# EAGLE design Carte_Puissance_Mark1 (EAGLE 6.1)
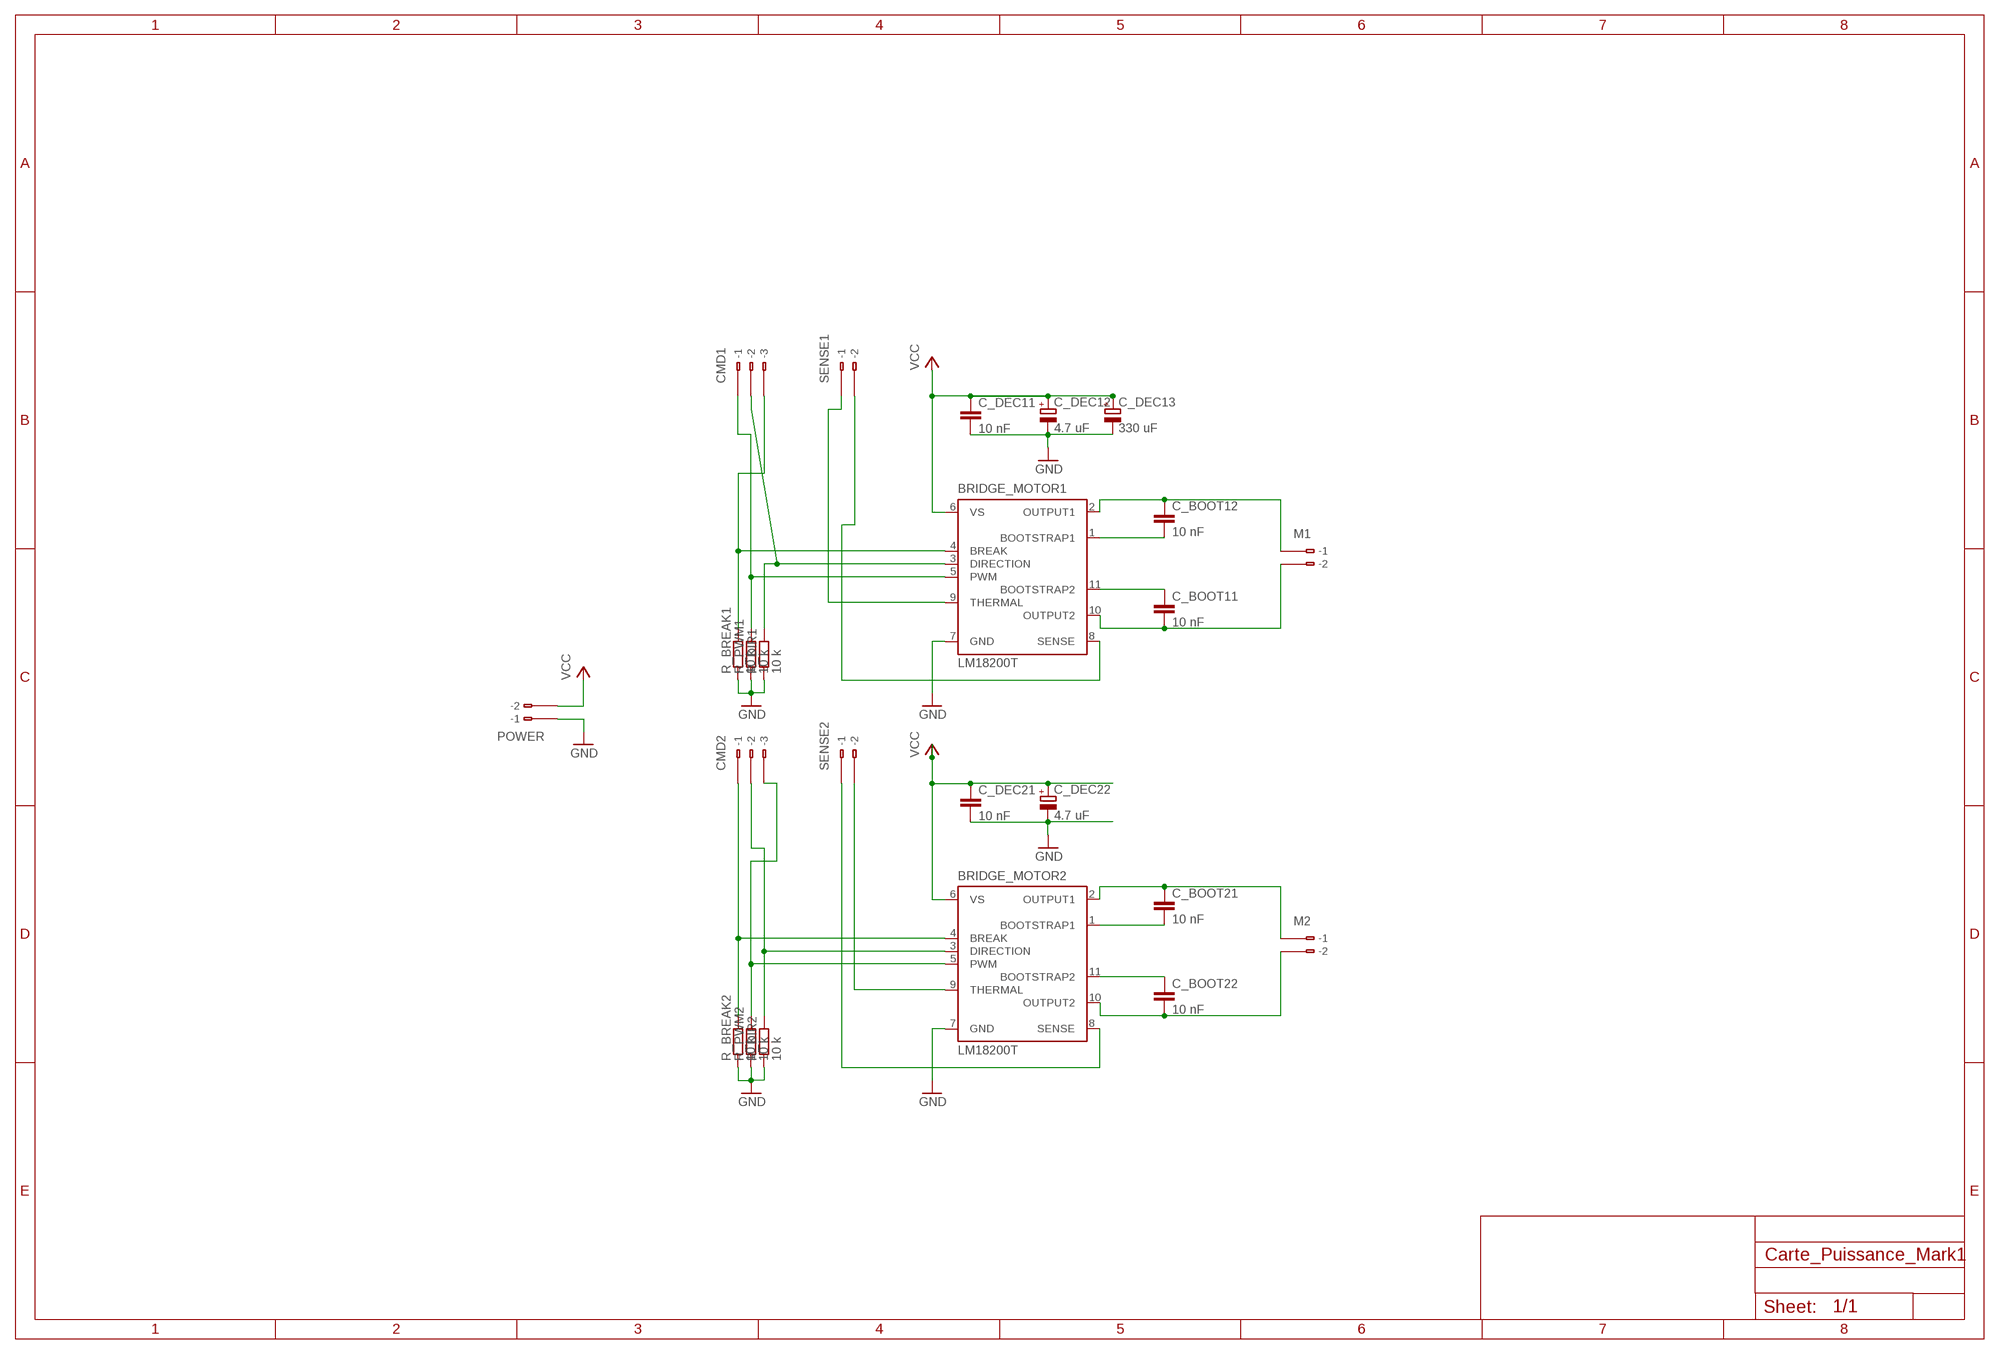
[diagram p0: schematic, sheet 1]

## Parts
BRIDGE_MOTOR1  LM18200T  [TO-220-11]
BRIDGE_MOTOR2  LM18200T  [TO-220-11]
C_BOOT11  10 nF  C5/3  [C5B3]
C_BOOT12  10 nF  C5/3  [C5B3]
C_BOOT21  10 nF  C5/3  [C5B3]
C_BOOT22  10 nF  C5/3  [C5B3]
C_DEC11  10 nF  C5/3  [C5B3]
C_DEC12  4.7 uF  CPOL-EUE2-5  [E2-5]
C_DEC13  330 uF  CPOL-EUE5-10.5  [E5-10,5]
C_DEC21  10 nF  C5/3  [C5B3]
C_DEC22  4.7 uF  CPOL-EUE2-5  [E2-5]
CMD1  233-103  [233-103]
CMD2  233-103  [233-103]
M1  233-102  [233-102]
M2  233-102  [233-102]
POWER  233-102  [233-102]
R_BREAK1  10 k  R-EU_R2012  [R2012]
R_BREAK2  10 k  R-EU_R2012  [R2012]
R_DIR1  10 k  R-EU_R2012  [R2012]
R_DIR2  10 k  R-EU_R2012  [R2012]
R_PWM1  10 k  R-EU_R2012  [R2012]
R_PWM2  10 k  R-EU_R2012  [R2012]
SENSE1  233-102  [233-102]
SENSE2  233-102  [233-102]

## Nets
GND: BRIDGE_MOTOR1.7(GND) BRIDGE_MOTOR2.7(GND) C_DEC11.2 C_DEC12.- C_DEC13.- C_DEC21.2 C_DEC22.- R_BREAK1.1 R_BREAK2.1 R_DIR1.1 R_DIR2.1 R_PWM1.1 R_PWM2.1
N$1: BRIDGE_MOTOR1.4(BREAK) CMD1.B3(B-3) R_BREAK1.2
N$2: BRIDGE_MOTOR1.5(PWM) CMD1.B1(B-1) R_PWM1.2
N$3: BRIDGE_MOTOR2.11(BOOTSTRAP2) C_BOOT22.1
N$4: BRIDGE_MOTOR2.1(BOOTSTRAP1) C_BOOT21.2
N$5: BRIDGE_MOTOR2.2(OUTPUT1) C_BOOT21.1 M2.B1(B-1)
N$6: BRIDGE_MOTOR2.10(OUTPUT2) C_BOOT22.2 M2.B2(B-2)
N$7: BRIDGE_MOTOR1.11(BOOTSTRAP2) C_BOOT11.1
N$8: BRIDGE_MOTOR1.1(BOOTSTRAP1) C_BOOT12.2
N$9: BRIDGE_MOTOR1.2(OUTPUT1) C_BOOT12.1 M1.B1(B-1)
N$10: BRIDGE_MOTOR1.10(OUTPUT2) C_BOOT11.2 M1.B2(B-2)
N$11: BRIDGE_MOTOR1.3(DIRECTION) CMD1.B2(B-2) R_DIR1.2
N$12: BRIDGE_MOTOR1.9(THERMAL) SENSE1.B1(B-1)
N$13: BRIDGE_MOTOR1.8(SENSE) SENSE1.B2(B-2)
N$14: BRIDGE_MOTOR2.4(BREAK) CMD2.B1(B-1) R_BREAK2.2
N$15: BRIDGE_MOTOR2.5(PWM) CMD2.B3(B-3) R_PWM2.2
N$16: BRIDGE_MOTOR2.3(DIRECTION) CMD2.B2(B-2) R_DIR2.2
N$17: BRIDGE_MOTOR2.9(THERMAL) SENSE2.B2(B-2)
N$18: BRIDGE_MOTOR2.8(SENSE) SENSE2.B1(B-1)
POWERT: POWER.B1(B-1) ; supply symbol labelled GND
VCC: BRIDGE_MOTOR1.6(VS) BRIDGE_MOTOR2.6(VS) C_DEC11.1 C_DEC12.+ C_DEC13.+ C_DEC21.1 C_DEC22.+ POWER.B2(B-2)
Unconnected: CMD1.A1(-1) CMD1.A2(-2) CMD1.A3(-3) CMD2.A1(-1) CMD2.A2(-2) CMD2.A3(-3) M1.A1(-1) M1.A2(-2) M2.A1(-1) M2.A2(-2) POWER.A1(-1) POWER.A2(-2) SENSE1.A1(-1) SENSE1.A2(-2) SENSE2.A1(-1) SENSE2.A2(-2)

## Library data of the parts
BRIDGE_MOTOR1 BRIDGE_MOTOR2 = national-semiconductor:LM18200T: 3A, 55V H-Bridge Motor Control SourcE: http://cache.national.com/ds/LM/LMD18200.pdf; OC_FARNELL: unknown; OC_NEWARK: unknown
C_BOOT11 C_BOOT12 C_BOOT21 C_BOOT22 C_DEC11 C_DEC21 = capacitor-wima:C: CAPACITOR
C_DEC12 C_DEC13 C_DEC22 = rcl:CPOL-EU: POLARIZED CAPACITOR, European symbol
CMD1 CMD2 = con-wago:233-103: WAGO Cage Clamp; MPN: 233-103; OC_FARNELL: unknown; OC_NEWARK: 28K9045
M1 M2 POWER SENSE1 SENSE2 = con-wago:233-102: WAGO Cage Clamp; MPN: 233-102; OC_FARNELL: unknown; OC_NEWARK: 28K9044
R_BREAK1 R_BREAK2 R_DIR1 R_DIR2 R_PWM1 R_PWM2 = resistor:R-EU_: RESISTOR, European symbol

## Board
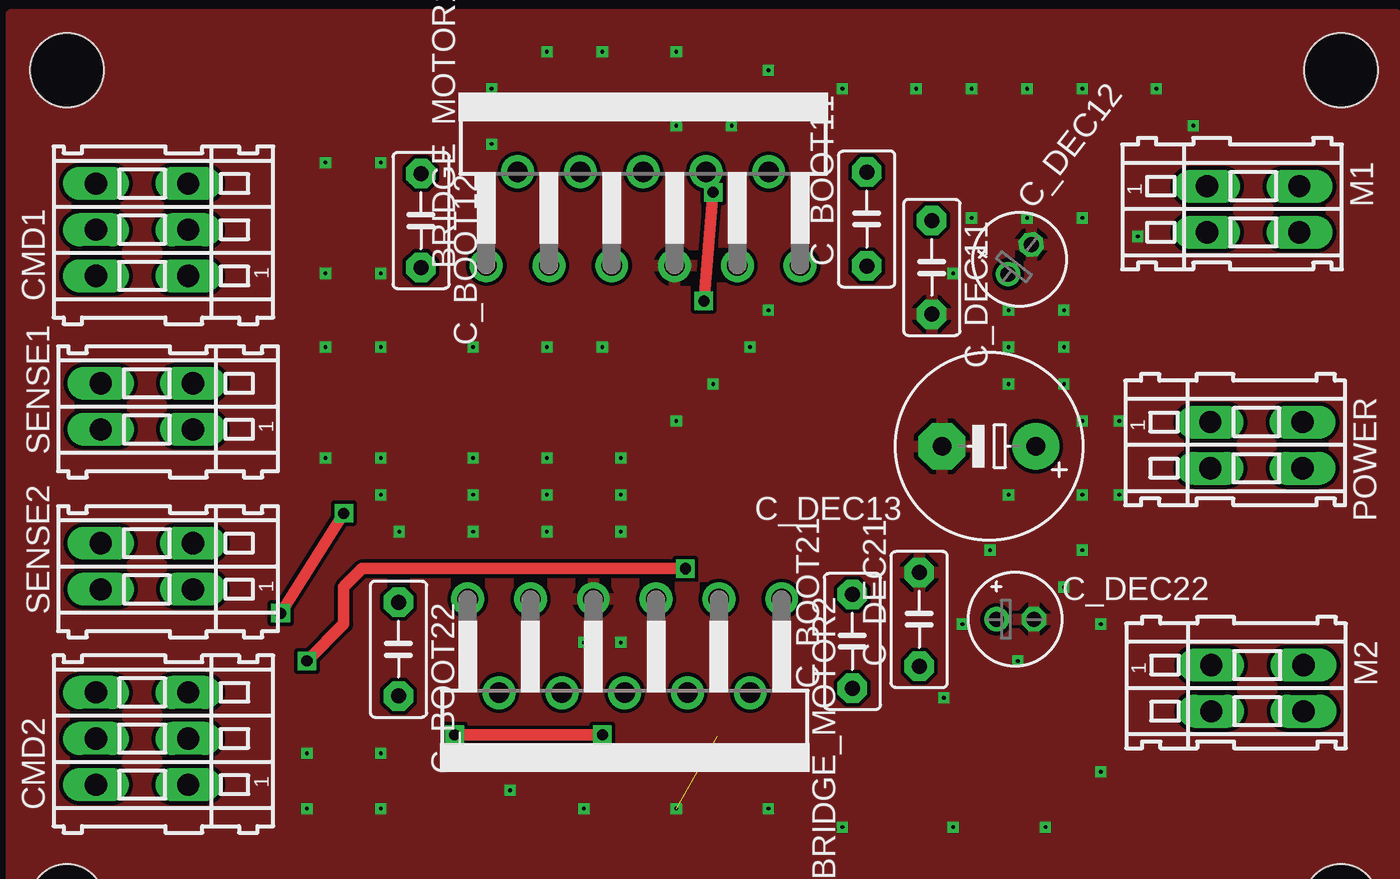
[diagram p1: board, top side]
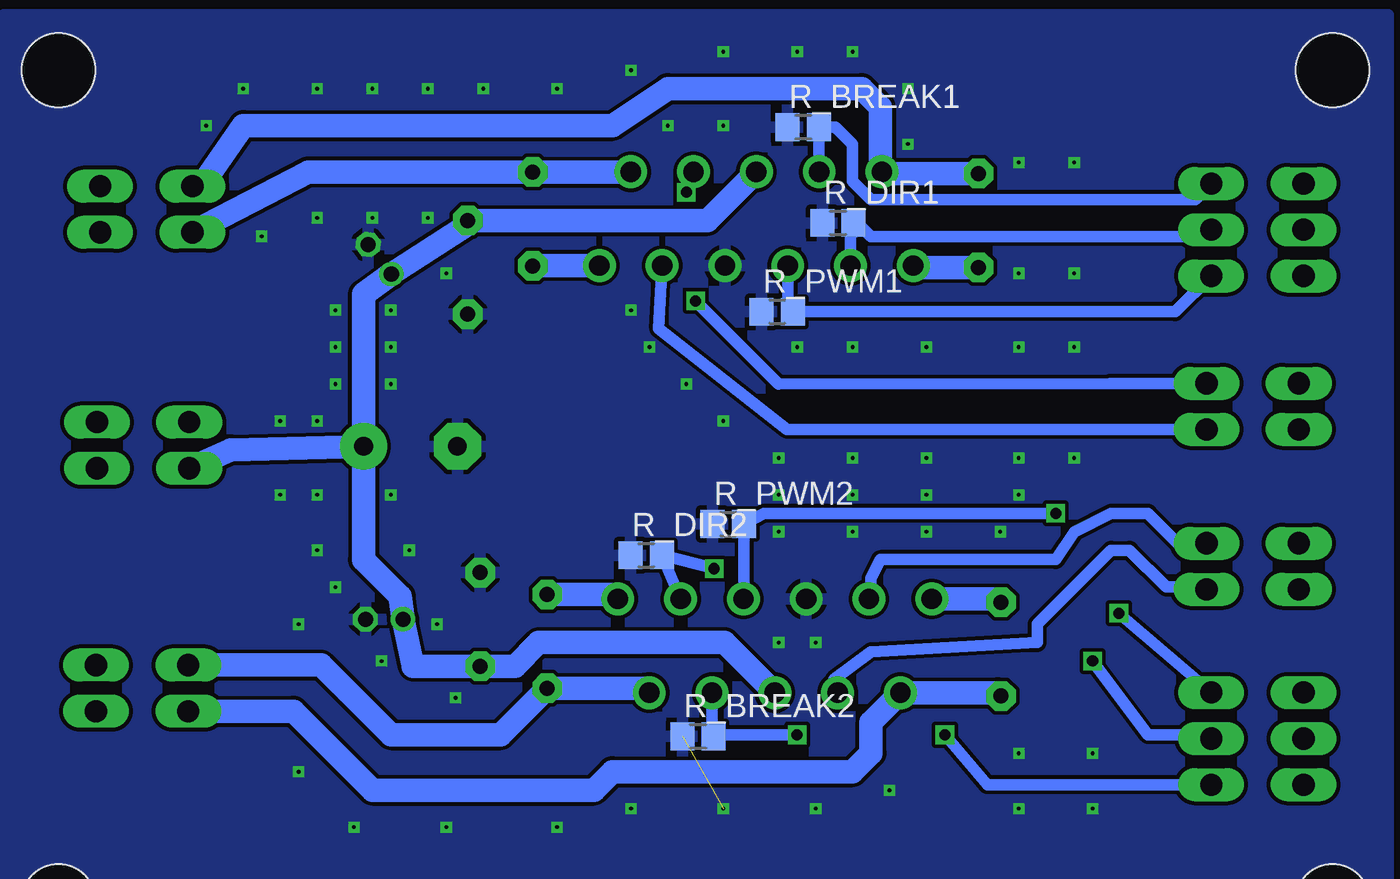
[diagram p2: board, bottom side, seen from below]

No outline drawn. Coordinates in mm, seen from the top.
Copper layers (1*16): Top 0.035mm / dielectric 1.5mm / Bottom 0.035mm
Design rules: minimum track width 10mil, minimum drill 1mil, track to track 8mil, track to pad 8mil, pad to pad 8mil, via to via 8mil, smd to smd 8mil, copper to edge 0mil, drill to drill 8mil, minimum pad ring 10mil, minimum via ring 8mil, stop-mask expansion 4mil, vias tented up to drill 0mil, thermal gap 10mil
Holes 4 mm at 3,49 72,49 72,4 3,4
tKeepout: area -2.1,43.9 to 8.1,54.1; area 66.9,43.9 to 77.1,54.1; area 66.9,-1.1 to 77.1,9.1; area -2.1,-1.1 to 8.1,9.1
bKeepout: area -2.1,43.9 to 8.1,54.1; area 66.9,43.9 to 77.1,54.1; area -2.1,-1.1 to 8.1,9.1; area 66.9,-1.1 to 77.1,9.1

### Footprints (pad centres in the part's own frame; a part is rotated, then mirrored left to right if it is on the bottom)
TO-220-11 = drill 1.1 pad 1.778: 1 -8.5,-9.37; 2 -6.8,-4.29; 3 -5.1,-9.37; 4 -3.4,-4.29; 5 -1.7,-9.37; 6 0,-4.29; 7 1.7,-9.37; 8 3.4,-4.29; 9 5.1,-9.37; 10 6.8,-4.29; 11 8.5,-9.37
C5B3 = drill 0.813 pad 1.6 octagon: 1 -2.54,0; 2 2.54,0
E2-5 = drill 0.813 pad 1.27: + -1.016,0 | drill 0.813 pad 1.27 octagon: - 1.016,0
E5-10,5 = drill 1.016 pad 2.54: + -2.54,0 | drill 1.016 pad 2.54 octagon: - 2.54,0
233-103 = drill 1.2 long: A1 -2.5,2.5; A2 0,2.5; A3 2.5,2.5; B1 -2.5,-2.5; B2 0,-2.5; B3 2.5,-2.5
233-102 = drill 1.2 long: A1 -1.25,2.5; A2 1.25,2.5; B1 -1.25,-2.5; B2 1.25,-2.5
R2012 = smd 1.3 x 1.5: 1 -0.85,0; 2 0.85,0

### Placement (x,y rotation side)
BRIDGE_MOTOR1  34.21,47.79 0 top
BRIDGE_MOTOR2  33.21,10.99 180 top
C_BOOT11  46.32,40.94 90 top
C_BOOT12  22.18,40.86 270 top
C_BOOT21  45.54,18.06 90 top
C_BOOT22  20.96,17.64 270 top
C_DEC11  49.84,38.32 270 top
C_DEC12  54.6,38.76 52.1 top
C_DEC13  52.94,28.63 180 top
C_DEC21  49.16,19.25 90 top
C_DEC22  54.36,19.26 0 top
CMD1  7.08,40.36 90 top
CMD2  7.08,12.8 90 top
M1  67.25,41.47 270 top
M2  67.47,15.53 270 top
POWER  67.42,28.69 270 top
R_BREAK1  31.67,45.92 0 bottom
R_BREAK2  37.37,12.92 0 bottom
R_DIR1  29.79,40.73 0 bottom
R_DIR2  40.18,22.73 0 bottom
R_PWM1  33.08,35.92 0 bottom
R_PWM2  35.74,24.42 0 bottom
SENSE1  7.33,30.79 90 top
SENSE2  7.33,22.13 90 top

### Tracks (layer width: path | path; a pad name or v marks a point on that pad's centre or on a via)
GND  (via drill 0.2)  (1 unrouted)
  Top 0.61: C_DEC11.2 49.84,35.84 50,36
  other vias: 29,26 33,26 25,26 20,26 59,11 56,8 51,8 45,8 41,9 36,9 31,9 27,10 59,19 54,26 53,23 51.5,19 58,23 58,26 57,21 58,30 57,36 57,34 57,32 54,32 54,34 54,36 51,38 52,41 58,41 55,41 58,48 55,48 52,48 62,48 61,40 64,46 49,48 45,48 41,49 36,50 32,50 29,50 26,48 26,45 20,28 25,28 29,28 33,28 20,34 25,34 29,34 32,34 20,38 17,34 17,38 17,44 20,44 20,9 16,9 16,12 20,12 17,28 60,30 60,26 36,46 39,46 36,30 38,32 40,34 41,36 50.5,15 54.5,17 33,24 29,24 25,24 21,24 31,18 33,18
  pour Top: 0,52 75,52 75,0 0,0
  pour Bottom: 0,52 75,52 75,0 0,0
N$1
  Bottom 0.61: BRIDGE_MOTOR1.4 R_BREAK1.2 29.92,45.92 29,45 29,43 28,42 10.44,42 CMD1.B3
N$2
  Bottom 0.61: BRIDGE_MOTOR1.5 32.51,36.2 R_PWM1.2 11.52,35.92 CMD1.B1
N$3
  Bottom 1.27: BRIDGE_MOTOR2.11 21.14,20.36 C_BOOT22.1
N$4
  Bottom 1.27: C_BOOT21.2 41.95,20.6 BRIDGE_MOTOR2.1
N$5
  Bottom 1.27: BRIDGE_MOTOR2.2 40.25,15.52 C_BOOT21.1 48.06,13 54,13 57.78,16.78 | 57.78,16.78 M2.B1 57.78,16.78
N$6
  Bottom 1.27: C_BOOT22.2 21.14,15.28 BRIDGE_MOTOR2.10 28,13.69 28,12 29,11 42,11 43,10 55,10 59.28,14.28 M2.B2
N$7
  Bottom 1.27: BRIDGE_MOTOR1.11 46.3,38.42 C_BOOT11.1
N$8
  Bottom 1.27: C_BOOT12.2 25.61,38.32 BRIDGE_MOTOR1.1
N$9
  Bottom 1.27: C_BOOT12.1 27.31,43.4 BRIDGE_MOTOR1.2 27.5,43.59 27.5,47 28.5,48 39,48 42,46 | M1.B1 64.28,42.72 62,46 | 62,46 42,46 | 62,46 42,46
N$10
  Bottom 1.27: BRIDGE_MOTOR1.10 41.03,43.48 C_BOOT11.2 58.49,43.48 M1.B2
N$11
  Bottom 0.61: BRIDGE_MOTOR1.3 29.11,40 | 29.11,40 29.11,40.89 29,41 28,40 9.94,40 CMD1.B2 | R_DIR1.2 28.94,40.17 29.11,40
N$12
  Bottom 0.61: SENSE1.B1 32.54,29.54 39.5,35 BRIDGE_MOTOR1.9
N$13  (via drill 0.6)
  Top 0.61: v37.5,36.5 v38,42.39
  Bottom 0.61: SENSE1.B2 15.04,32.04 | v38,42.39 BRIDGE_MOTOR1.8 | v37.5,36.5 33,32 | 33,32 15.04,32.04 | 33,32 15.04,32.04
N$14  (via drill 0.6)
  Top 0.61: v24,13 v32,13
  Bottom 0.61: BRIDGE_MOTOR2.4 36.61,13.01 R_BREAK2.2 36.44,13 v32,13 | CMD2.B1 21.7,10.3 v24,13
N$15  (via drill 0.6)
  Top 0.61: v14.58,19.58 v18,25
  Bottom 0.61: BRIDGE_MOTOR2.5 34.89,20.38 R_PWM2.2 33.81,25 v18,25 | CMD2.B3 v14.58,19.58
N$16  (via drill 0.6)
  Top 0.61: v16,17 18,19 18,21 19,22 v36.5,22
  Bottom 0.61: BRIDGE_MOTOR2.3 R_DIR2.2 39.23,22.73 v36.5,22 | CMD2.B2 10.78,13 13,13 v16,17
N$17
  Bottom 0.61: SENSE2.B2 11.38,23.38 13,25 15,25 17,24 18,22.5 27.5,22.5 28,21.5 28,20.47 BRIDGE_MOTOR2.9
N$18
  Bottom 0.61: BRIDGE_MOTOR2.8 30,15.47 30,16 28,17.5 19,18 19,19 15,23 14,23 12,21 9.95,21 SENSE2.B1
VCC
  Bottom 1.27: BRIDGE_MOTOR1.6 36.85,40.86 C_DEC11.1 49.48,40.86 C_DEC12.+ 55.48,36.86 C_DEC13.+ | BRIDGE_MOTOR2.6 35.93,18 46,18 47.29,16.71 C_DEC21.1 52.79,16.71 C_DEC22.+ 53.5,20.5 55.48,22.48 | POWER.B2 62.67,28.44 C_DEC13.+ | C_DEC13.+ 55.48,22.48 | C_DEC13.+ 55.48,22.48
